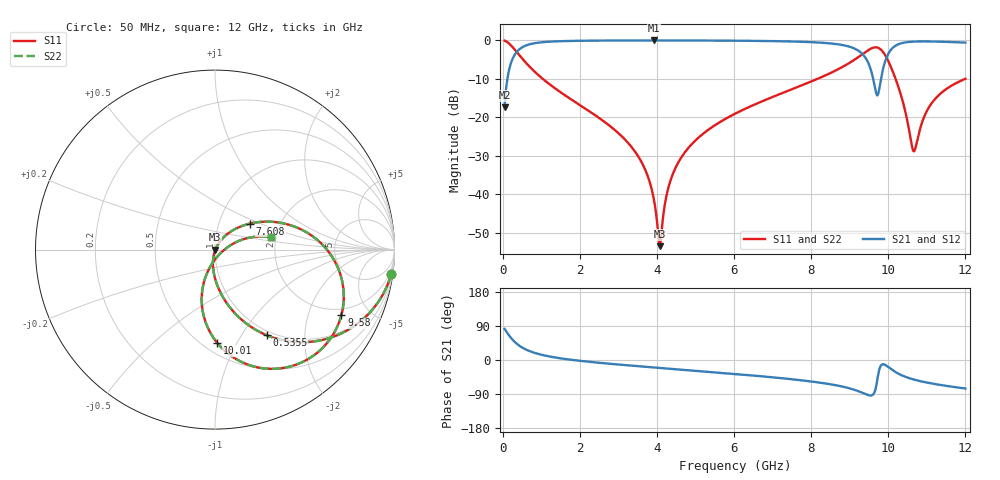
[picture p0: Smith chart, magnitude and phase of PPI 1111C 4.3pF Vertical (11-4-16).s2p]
# GHz S MA R 50
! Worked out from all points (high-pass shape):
!   1601 points, 50 MHz to 12 GHz, reference 50 ohm
!   highest |S21| = -0.02 dB at 3.934 GHz (marker M1); lowest = -17.4 dB at 50 MHz (marker M2)
!   |S21| within 3 dB of the highest: 363 MHz to 9.272 GHz (8.909 GHz wide, 185 % of centre); 10.03 GHz to end of sweep
!   lowest |S11| = -53.5 dB at 4.076 GHz (marker M3), VSWR 1.00, Z = 50.2 - j0.0707 ohm
!   |S11| at or under -10 dB: 1.039 GHz to 8.165 GHz (7.126 GHz wide, 155 % of centre); 10.19 GHz to 12 GHz (1.808 GHz wide, 16.3 % of centre)
!   |S22| runs from -53.5 to -0.1 dB; largest |S21 - S12| = 0
!   S11 on the Smith chart (normalised r, x): 50 MHz: 1, -14; 535.5 MHz: 0.94, -1.30; 7.608 GHz: 1.41, +0.43; 9.58 GHz: 1.68, -3.31; 10.01 GHz: 0.59, -0.84; 12 GHz: 1.87, +0.28
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0.05  0.9908 -8.0  0.1355 82.0  0.1355 82.0  0.9908 -8.0
0.22925  0.8466 -33.3  0.5319 56.6  0.5319 56.6  0.8466 -33.3
0.5354688  0.5584 -58.8  0.8288 31.2  0.8288 31.2  0.5584 -58.8
1.043344  0.3149 -76.9  0.948 12.9  0.948 12.9  0.3149 -76.9
2.044156  0.1396 -92.0  0.9887 -2.6  0.9887 -2.6  0.1396 -92.0
3.388531  0.03835 -102.5  0.9972 -15.3  0.9972 -15.3  0.03835 -102.5
3.732094  0.01882 -102.1  0.9976 -18.1  0.9976 -18.1  0.01882 -102.1
3.93375  0.007906 -94.7  0.9977 -19.8  0.9977 -19.8  0.007906 -94.7
4.038312  0.002871 -63.8  0.9977 -20.6  0.9977 -20.6  0.002871 -63.8
4.075656  0.002108 -19.5  0.9976 -20.9  0.9976 -20.9  0.002108 -19.5
4.299719  0.01229 57.0  0.9975 -22.7  0.9975 -22.7  0.01229 57.0
4.605937  0.02861 60.2  0.997 -25.2  0.997 -25.2  0.02861 60.2
6.025  0.1112 51.5  0.9903 -36.9  0.9903 -36.9  0.1112 51.5
7.608375  0.2432 36.6  0.9637 -52.0  0.9637 -52.0  0.2432 36.6
8.019156  0.2946 31.6  0.9473 -56.9  0.9473 -56.9  0.2946 31.6
9.094656  0.5483 7.9  0.7947 -77.7  0.7947 -77.7  0.5483 7.9
9.580125  0.7933 -27.4  0.3629 -93.0  0.3629 -93.0  0.7933 -27.4
9.7295  0.8038 -48.2  0.1961 -43.8  0.1961 -43.8  0.8038 -48.2
10.01331  0.5204 -88.6  0.6877 -19.5  0.6877 -19.5  0.5204 -88.6
10.66309  0.0361 -44.5  0.9636 -51.6  0.9636 -51.6  0.0361 -44.5
11.13363  0.1543 20.2  0.9669 -62.1  0.9669 -62.1  0.1543 20.2
12  0.3167 12.4  0.9352 -75.2  0.9352 -75.2  0.3167 12.4
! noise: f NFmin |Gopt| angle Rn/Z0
0.05  0.0004631  0.9067  2.634  0.001089
1.372  0.003977  0.6901  8.1  0.002485
2.701  0.006546  0.6425  14.45  0.003411
4.031  0.00898  0.6217  20.71  0.004297
5.36  0.01164  0.6201  26.79  0.005423
6.682  0.01529  0.6436  32.69  0.007506
8.012  0.02389  0.7221  38.8  0.01521
9.341  0.1046  0.9201  45.47  0.2464
10.67  0.0556  0.8408  51.34  0.06025
12  0.03562  0.7456  55.93  0.02208
